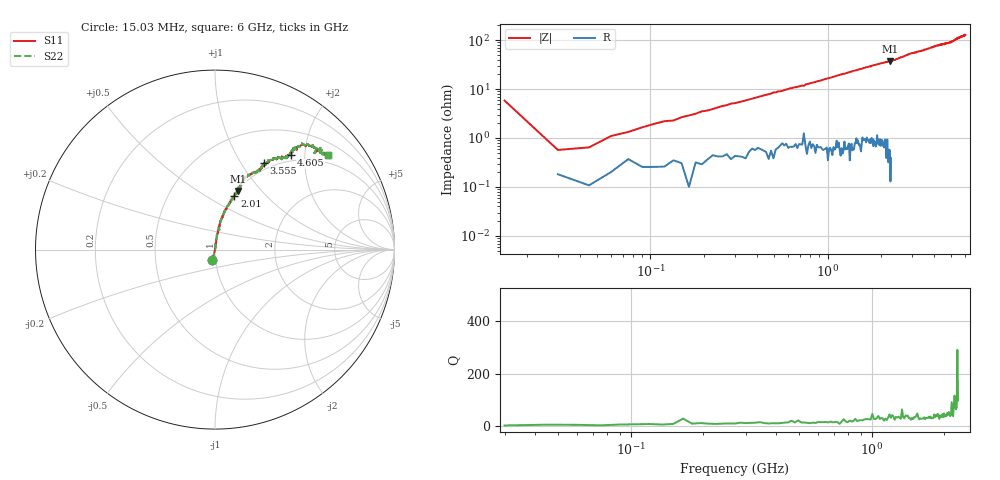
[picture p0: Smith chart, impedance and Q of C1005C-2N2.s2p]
!	Network	Analyzer	HP8753E.07.74:	Oct	30	2002	Serial	No.	JP38451487
!	Hewlett-Packard
!	7	Sep	2009	8:17:41
!	Frequency	S11	S21	S12	S22
#	HZ	S	RI	R	50
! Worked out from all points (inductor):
!   400 points, 15.03 MHz to 6 GHz, reference 50 ohm
!   read as one part in series: L = 2.71 nH near 45.03 MHz
!   highest Q = 83.1 at 2.25 GHz (marker M1), where L = 2.66 nH
!   S11 on the Smith chart (normalised r, x): 15.03 MHz: 0.97, -0.11; 2.01 GHz: 1.02, +0.67; 3.555 GHz: 0.91, +1.27; 4.605 GHz: 0.89, +1.73; 6 GHz: 0.79, +2.54
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1.502992e7  -0.0143 -0.0576  1.01 0.0576  1.01 0.0576  -0.0143 -0.0576
3.002985e7  0.0017 0.0054  0.998 -0.0054  0.998 -0.0054  0.0017 0.0054
4.502978e7  0.00124 0.00634  0.999 -0.00634  0.999 -0.00634  0.00124 0.00634
6.00297e7  0.00228 0.0108  0.998 -0.0108  0.998 -0.0108  0.00228 0.0108
1.050295e8  0.00288 0.0192  0.997 -0.0192  0.997 -0.0192  0.00288 0.0192
1.95029e8  0.00421 0.0347  0.996 -0.0347  0.996 -0.0347  0.00421 0.0347
2.850286e8  0.00639 0.0498  0.994 -0.0498  0.994 -0.0498  0.00639 0.0498
4.950275e8  0.011 0.0842  0.989 -0.0842  0.989 -0.0842  0.011 0.0842
1.020025e9  0.0332 0.162  0.967 -0.162  0.967 -0.162  0.0332 0.162
1.395023e9  0.0574 0.22  0.943 -0.22  0.943 -0.22  0.0574 0.22
2.01002e9  0.108 0.297  0.892 -0.297  0.892 -0.297  0.108 0.297
2.250019e9  0.127 0.326  0.873 -0.326  0.873 -0.326  0.127 0.326
3.015015e9  0.219 0.431  0.781 -0.431  0.781 -0.431  0.219 0.431
3.555012e9  0.274 0.484  0.726 -0.484  0.726 -0.484  0.274 0.484
4.00501e9  0.35 0.515  0.65 -0.515  0.65 -0.515  0.35 0.515
4.575007e9  0.394 0.516  0.606 -0.516  0.606 -0.516  0.394 0.516
4.605007e9  0.424 0.526  0.576 -0.526  0.576 -0.526  0.424 0.526
5.010005e9  0.453 0.568  0.547 -0.568  0.547 -0.568  0.453 0.568
5.175004e9  0.484 0.592  0.516 -0.592  0.516 -0.592  0.484 0.592
5.445003e9  0.567 0.564  0.433 -0.564  0.433 -0.564  0.567 0.564
5.535002e9  0.552 0.537  0.448 -0.537  0.448 -0.537  0.552 0.537
6e9  0.63 0.526  0.37 -0.526  0.37 -0.526  0.63 0.526
